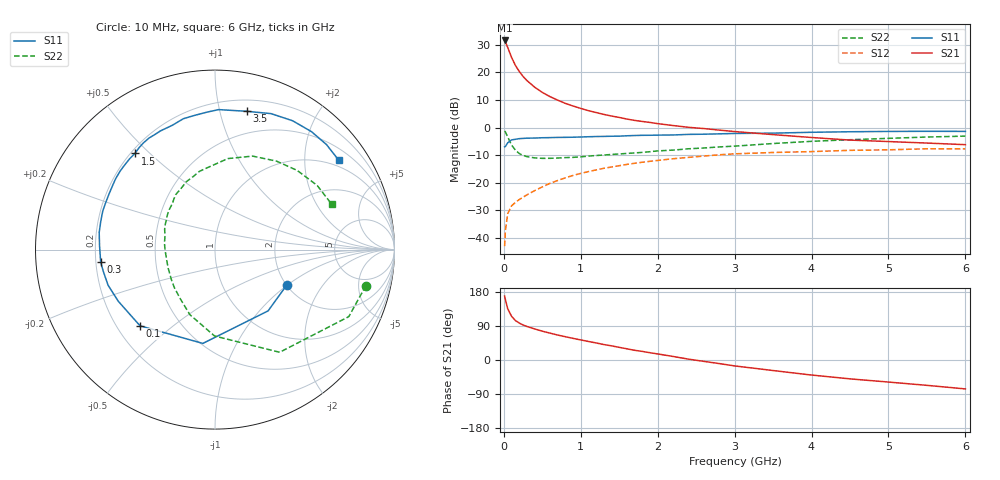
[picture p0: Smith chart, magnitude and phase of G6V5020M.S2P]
! SIEMENS Small Signal Semiconductors
! BFG193
! Si NPN RF Bipolar Junction Transistor in SOT223
! VCE = 0.5 V  IC = 20 mA
! Common Emitter S-Parameters:  August  1996
# GHz  S  MA  R  50
!  f  S11  S21  S12  S22
! GHz  MAG  ANG  MAG  ANG  MAG  ANG  MAG  ANG
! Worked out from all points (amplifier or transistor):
!   36 points, 10 MHz to 6 GHz, reference 50 ohm
!   highest |S21| = 31.6 dB at 10 MHz (marker M1)
!   |S21| within 3 dB of that: start of sweep to 56.64 MHz
!   unconditionally stable (mu >= 1): 468.3 MHz to end of sweep
!   at 250 MHz: K = 0.80, MSG = 21.9 dB, |S12| = -25.3 dB
!   at 1.4 GHz: K = 1.11, MAG = 7.2 dB, |S12| = -14.3 dB
!   at 6 GHz: K = 1.02, MAG = -0.1 dB, |S12| = -7.8 dB
!   S11 on the Smith chart (normalised r, x): 10 MHz: 2.02, -0.99; 100 MHz: 0.29, -0.39; 300 MHz: 0.22, -0.05; 1.5 GHz: 0.22, +0.45; 3.5 GHz: 0.30, +1.21; 6 GHz: 0.80, +2.90
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0.01  0.4464 -26.0  38.13 168.8  0.007 80.7  0.8644 -13.4
0.02  0.4518 -49.1  36.23 159.4  0.0134 74.9  0.8338 -26.6
0.05  0.5271 -97.4  28.52 135.4  0.0272 57.0  0.676 -57.8
0.1  0.5956 -134.5  18.83 115.5  0.0377 47.3  0.4813 -90.3
0.15  0.6109 -151.9  13.46 104.2  0.0438 45.6  0.3887 -111.1
0.2  0.628 -161.6  10.46 97.5  0.0491 46.4  0.3375 -124.4
0.25  0.634 -169.0  8.463 92.4  0.0543 48.3  0.311 -136.5
0.3  0.6408 -173.7  7.133 88.5  0.0599 49.5  0.2963 -144.6
0.4  0.6436 178.1  5.412 82.0  0.0713 51.5  0.2808 -158.1
0.5  0.6522 171.6  4.344 76.1  0.0835 52.0  0.2754 -168.0
0.6  0.6557 166.1  3.64 70.9  0.0969 52.1  0.2759 -175.4
0.7  0.6613 161.0  3.14 65.9  0.1091 51.6  0.2795 178.3
0.8  0.6629 156.5  2.745 61.4  0.1219 50.3  0.2843 172.2
1.1  0.68 144.5  2.024 48.9  0.1584 45.8  0.3026 158.0
1.5  0.6971 129.8  1.525 33.4  0.2026 36.9  0.331 142.6
1.7  0.7157 123.9  1.346 25.6  0.2241 32.8  0.3455 134.7
2.2  0.7324 108.9  1.087 9.3  0.271 20.4  0.389 119.3
3  0.7802 88.5  0.845 -15.6  0.3328 1.3  0.4589 95.1
3.5  0.7908 77.0  0.743 -27.8  0.3521 -11.6  0.512 82.0
4.5  0.8381 58.9  0.591 -49.8  0.3853 -30.3  0.6004 55.2
5.5  0.8534 43.3  0.522 -66.9  0.4115 -51.8  0.6721 32.2
6  0.8506 35.8  0.488 -76.3  0.4083 -64.0  0.6978 21.2
